|Texas Instruments Incorporated
| Marketing part#   Digital Voltage Range   Package-type   #pins
|24-Channel, Constant-Current LED Driver with
|   Global Brightness Control and LED Open-Short Detection
| TLC5951DAP   3.0V - 5.5V   HTSSOP   32
| TLC5951DAPR   3.0V - 5.5V   HTSSOP   32
| TLC5951RHAR   3.0V - 5.5V   VQFN   40
| TLC5951RHAT   3.0V - 5.5V   VQFN   40
|24-Channel Constant-Current LED Driver with Global Brightness and
|   LED Open Short Detection
| TLC5952DAP   3.0V - 5.5V   HTSSOP   32
| TLC5952DAPR   3.0V - 5.5V   HTSSOP   32
[IBIS Ver]   3.2
[File name]   tlc5951_2.ibs
|SIMDE Ver   V2.1 - 201006 - RHL4 - Build 390
[File Rev]   1.0
[Date]   9/23/2010
[Source]
| Texas Instruments Incorporated.
| Analog-eLab Design Center, HPA
| 12500 TI Blvd
| Dallas, TX -75243
| e-mail: elab_ibis@list.ti.com
| -Model generated from simulations in TISPICE
[Notes]   Revision History:
| Rev 1.0: 9/23/2010
| - Initial version of the model
| - Model generated from simulations in TISPICE
| - Model matched to SPICE simulation
| - C_comp although listed in numerical order of value are
|   obtained from varying PVT conditions. For PVT conditions for
|   each specific value refer the buffer description under
|   respective [Model]. IBIS model user is responsible for using
|   appropriate C_comp to simulate for Signal Integrity.
| Rev 2.0: 11/09/2010
| - Added TLC5951 to this file.
[Disclaimer]
| This model is designed as an aid for customers of Texas Instruments.
| TI and its licensors and suppliers make no warranties, either expressed
| or implied, with respect to this  model, including the warranties of
| merchantability or fitness for a particular purpose. The model is
| provided solely on an "as is" basis. The entire risk as to its quality
| and performance is with the customer.
[Copyright]
 (C) Copyright 2010 Texas Instruments Incorporated.All rights reserved.
|   TLC5951
[Component]   tlc5951dap
[Manufacturer]   TI
[Package]   |38 TSSOP -  DAP package
|   typ   min   max
R_pkg   8.17672E-02   6.24500E-02   1.08010E-01
L_pkg   2.92970E+00nH 2.04966E+00nH 4.47905E+00nH
C_pkg   4.58117E-01pF 3.25640E-01pF 7.17190E-01pF
[Pin]  signal_name   model_name   R_pin   L_pin   C_pin
1   GSSIN   INPUT1   0.09315  4.34776nH  0.70829pF
2   GSSCK   INPUT1   0.09141  3.78923nH  0.64273pF
3   GSLAT   INPUT1   0.09208  3.37817nH  0.51017pF
4   GSCKG   INPUT1   0.09705  3.12890nH  0.41894pF
5   GSCKR   INPUT1   0.07908  2.56520nH  0.38281pF
6   GSCKB   INPUT1   0.06932  2.29870nH  0.38677pF
7   OUTG0   TERM   0.07284  2.36160nH  0.39548pF
8   OUTR0   TERM   0.06720  2.20089nH  0.35323pF
9   OUTB0   TERM   0.06392  2.10626nH  0.32825pF
10   OUTG1   TERM   0.06245  2.04966nH  0.33776pF
11   OUTR1   TERM   0.06251  2.07259nH  0.32616pF
12   OUTB1   TERM   0.06454  2.13381nH  0.35151pF
13   OUTG2   TERM   0.06899  2.26419nH  0.40004pF
14   OUTR2   TERM   0.07658  2.47960nH  0.40706pF
15   OUTB2   TERM   0.08918  2.79631nH  0.39459pF
16   OUTG3   TERM   0.10801  3.42213nH  0.43527pF
17   OUTR3   TERM   0.09962  3.58013nH  0.52374pF
18   OUTB3   TERM   0.09131  3.79687nH  0.63821pF
19   GSSOUT   OUTPUT   0.09415  4.38631nH  0.70306pF
20   DCSOUT   OUTPUT   0.09412  4.38435nH  0.70183pF
21   OUTB4   TERM   0.09133  3.79971nH  0.63660pF
22   OUTR4   TERM   0.09967  3.58487nH  0.52283pF
23   OUTG4   TERM   0.10780  3.37452nH  0.42376pF
24   OUTB5   TERM   0.08925  2.80655nH  0.39086pF
25   OUTR5   TERM   0.07653  2.45754nH  0.38662pF
26   OUTG5   TERM   0.06903  2.27056nH  0.39766pF
27   OUTB6   TERM   0.06456  2.13669nH  0.35087pF
28   OUTR6   TERM   0.06253  2.07560nH  0.32564pF
29   OUTG6   TERM   0.06246  2.05175nH  0.33765pF
30   OUTB7   TERM   0.06393  2.10761nH  0.32820pF
31   OUTR7   TERM   0.06717  2.19528nH  0.35713pF
32   OUTG7   TERM   0.07282  2.35785nH  0.40264pF
33   GND   GND   0.02545  1.83237nH  0.44923pF
34   IREF   TERM   0.07803  2.57211nH  0.38528pF
35   VCC   POWER   0.10133  3.23896nH  0.42035pF
36   XBLNK   INPUT2   0.10289  3.65360nH  0.52550pF
37   DCSCK   INPUT1   0.09983  4.00327nH  0.65787pF
38   DCSIN   INPUT1   0.09828  4.47905nH  0.71719pF
|   TLC5951
[Component]   tlc5951rha
[Manufacturer]   TI
[Package]   |40 VQFN -  RHA package
|   typ   min   max
R_pkg   9.32975E-02   6.33100E-02   1.19040E-01
L_pkg   1.59676E+00nH 1.06106E+00nH 2.06268E+00nH
C_pkg   1.89299E-01pF 1.56590E-01pF 2.16790E-01pF
[Pin]  signal_name   model_name   R_pin   L_pin   C_pin
1   OUTG3   TERM   0.10712  1.86107nH  0.19519pF
2   OUTR3   TERM   0.08648  1.47581nH  0.18946pF
3   OUTB3   TERM   0.06847  1.15145nH  0.16480pF
4   NC   NC   0.00070  0.13786nH  0.10009pF
5   GSSOUT   OUTPUT   0.06331  1.06106nH  0.15660pF
6   DCSOUT   OUTPUT   0.06331  1.06107nH  0.15659pF
7   NC   NC   0.00070  0.13788nH  0.10006pF
8   OUTB4   TERM   0.06847  1.15146nH  0.16478pF
9   OUTR4   TERM   0.08648  1.47583nH  0.18943pF
10   OUTG4   TERM   0.10712  1.86107nH  0.19518pF
11   OUTB5   TERM   0.11482  1.99637nH  0.19891pF
12   OUTR5   TERM   0.10670  1.83978nH  0.20708pF
13   OUTG5   TERM   0.10070  1.72764nH  0.19868pF
14   OUTB6   TERM   0.09716  1.66145nH  0.19427pF
15   OUTR6   TERM   0.09640  1.64661nH  0.19331pF
16   OUTG6   TERM   0.09851  1.68432nH  0.19584pF
17   OUTB7   TERM   0.10326  1.77105nH  0.20167pF
18   OUTR7   TERM   0.11026  1.89965nH  0.21014pF
19   OUTG7   TERM   0.11904  2.06267nH  0.21679pF
20   GND   GND   0.03821  1.46001nH  0.25096pF
21   IREF   TERM   0.09701  1.66907nH  0.18547pF
22   VCC   POWER   0.08821  1.50141nH  0.19349pF
23   XBLNK   INPUT2   0.08305  1.40645nH  0.18423pF
24   DCSCK   INPUT1   0.07318  1.22796nH  0.17357pF
25   DCSIN   INPUT1   0.06669  1.11239nH  0.16310pF
26   GSSIN   INPUT1   0.07184  1.20404nH  0.16885pF
27   GSSCK   INPUT1   0.06604  1.10089nH  0.16504pF
28   GSLAT   INPUT1   0.06725  1.12256nH  0.16630pF
29   GSCKG   INPUT1   0.08046  1.35982nH  0.18570pF
30   GSCKR   INPUT1   0.09935  1.71110nH  0.19097pF
31   GSCKB   INPUT1   0.10938  1.89107nH  0.18848pF
32   OUTG0   TERM   0.11904  2.06268nH  0.21453pF
33   OUTR0   TERM   0.11026  1.89964nH  0.21001pF
34   OUTB0   TERM   0.10326  1.77105nH  0.20165pF
35   OUTG1   TERM   0.09851  1.68430nH  0.19585pF
36   OUTR1   TERM   0.09640  1.64660nH  0.19331pF
37   OUTB1   TERM   0.09716  1.66144nH  0.19428pF
38   OUTG2   TERM   0.10070  1.72763nH  0.19869pF
39   OUTR2   TERM   0.10670  1.83977nH  0.20709pF
40   OUTB2   TERM   0.11482  1.99636nH  0.19893pF
|   TLC5952
[Component]   tlc5952dap
[Manufacturer]   TI
[Package]   |32 HTSSOP -  DAP package
|   typ   min   max
R_pkg   0.12967   0.11257   0.15633
L_pkg   3.26276nH   2.52801nH   4.32090nH
C_pkg   0.50954pF   0.38287pF   0.72149pF
[Pin]  signal_name   model_name   R_pin   L_pin   C_pin
1   GND   GND   0.04974   3.78413nH  0.77752pF
2   SIN   INPUT1   0.11858   3.73893nH  0.68715pF
3   SCLK   INPUT1   0.11836   3.34620nH  0.60838pF
4   LAT   INPUT2   0.13633   3.35082nH  0.52440pF
5   OUTR0   TERM   0.14689   3.16195nH  0.41891pF
6   OUTG0   TERM   0.12988   2.85912nH  0.40302pF
7   OUTB0   TERM   0.11839   2.62965nH  0.38972pF
8   OUTR1   TERM   0.11257   2.52801nH  0.38289pF
9   OUTG1   TERM   0.11445   2.56250nH  0.38511pF
10   OUTB1   TERM   0.12368   2.72726nH  0.39620pF
11   OUTR2   TERM   0.13760   3.00248nH  0.41278pF
12   OUTG2   TERM   0.15633   3.33801nH  0.42947pF
13   OUTB2   TERM   0.14744   3.63051nH  0.53993pF
14   OUTR3   TERM   0.13599   3.71934nH  0.65070pF
15   OUTG3   TERM   0.12663   3.93372nH  0.70742pF
16   OUTB3   TERM   0.12184   4.32090nH  0.72149pF
17   OUTR4   TERM   0.12109   4.22139nH  0.71128pF
18   OUTG4   TERM   0.12636   3.88596nH  0.70297pF
19   OUTB4   TERM   0.13607   3.66977nH  0.63027pF
20   OUTR5   TERM   0.14909   3.58859nH  0.53819pF
21   OUTG5   TERM   0.15633   3.33826nH  0.43057pF
22   OUTB5   TERM   0.13760   3.00263nH  0.41276pF
23   OUTR6   TERM   0.12368   2.72745nH  0.39613pF
24   OUTG6   TERM   0.11445   2.56257nH  0.38509pF
25   OUTB6   TERM   0.11257   2.52807nH  0.38287pF
26   OUTR7   TERM   0.11839   2.62965nH  0.38967pF
27   OUTG7   TERM   0.12988   2.85913nH  0.40268pF
28   OUTB7   TERM   0.14689   3.16169nH  0.41575pF
29   BLANK   INPUT1   0.12636   3.17477nH  0.50902pF
30   SOUT   OUTPUT   0.12223   3.41530nH  0.60971pF
31   VCC   POWER   0.12298   3.81745nH  0.69127pF
32   IREF   TERM   0.12422   4.26806nH  0.71157pF
|   Model Selectors
[Model Selector] INPUT1
SIN_SCLK_BLANK_3p3v   3.3V digital input
SIN_SCLK_BLANK_5p0v   5.0V digital input
|NOTES   Model INPUT1 split into two Models SIN_SCLK_BLANK_3p3v
|   and SIN_SCLK_BLANK_5p0v to accomodate vast voltage range
|   of 3.0V - 5.5V
|   SIN_SCLK_BLANK_3p3v operates in voltage range of 3.0 - 3.3 - 3.6
|   SIN_SCLK_BLANK_5p0v operates in voltage range of 4.5 - 5.0 - 5.5
[Model Selector] INPUT2
LAT_3p3v   3.3V digital input
LAT_5p0v   5.0V digital input
|NOTES   Model INPUT2 split into two Models LAT_3p3v
|   and LAT_5p0v to accomodate vast voltage range of 3.0V - 5.5V
|   LAT_3p3v operates in voltage range of 3.0 - 3.3 - 3.6
|   LAT_5p0v operates in voltage range of 4.5 - 5.0 - 5.5
[Model Selector] OUTPUT
SOUT_3p3v   3.3V digital input
SOUT_5p0v   5.0V digital input
|NOTES   Model OUTPUT split into two Models SOUT_3p3v
|   and SOUT_5p0v to accomodate vast voltage range of 3.0V - 5.5V
|   SOUT_3p3v operates in voltage range of 3.0 - 3.3 - 3.6
|   SOUT_5p0v operates in voltage range of 4.5 - 5.0 - 5.5
[Model Selector] TERM
TERM_3p3  3.3V nominal termination
TERM_5p0  5.0V nominal termination
|   TERM 3.3V Model
[Model]  TERM_3p3
Model_type Terminator
C_comp   1.0e-20F  1.0e-20F  1.0e-20F
|   typ   min   max
[Voltage Range]   3.3V   3.0V   3.6V
[POWER Clamp Reference]   3.3V   3.0V   3.6V
[GND Clamp Reference]   0V   0V   0V
|Ambient Temperature   25   85   -40
|Junction Temperature
[Temperature Range]   65   125   -40
|   TERM 5.0V Model
[Model]  TERM_5p0
Model_type Terminator
C_comp   1.0e-20F  1.0e-20F  1.0e-20F
|   typ   min   max
[Voltage Range]   5.0V   4.5V   5.5V
[POWER Clamp Reference]   5.0V   4.5V   5.5V
[GND Clamp Reference]   0V   0V   0V
|Ambient Temperature   25   85   -40
|Junction Temperature
[Temperature Range]   65   125   -40
| Models and submodels in the file (8): LAT_3p3v (Input), LAT_5p0v (Input), SIN_SCLK_BLANK_3p3v (Input), SIN_SCLK_BLANK_5p0v (Input), SOUT_3p3v (Output), SOUT_5p0v (Output), TERM_3p3 (Terminator), TERM_5p0 (Terminator)
